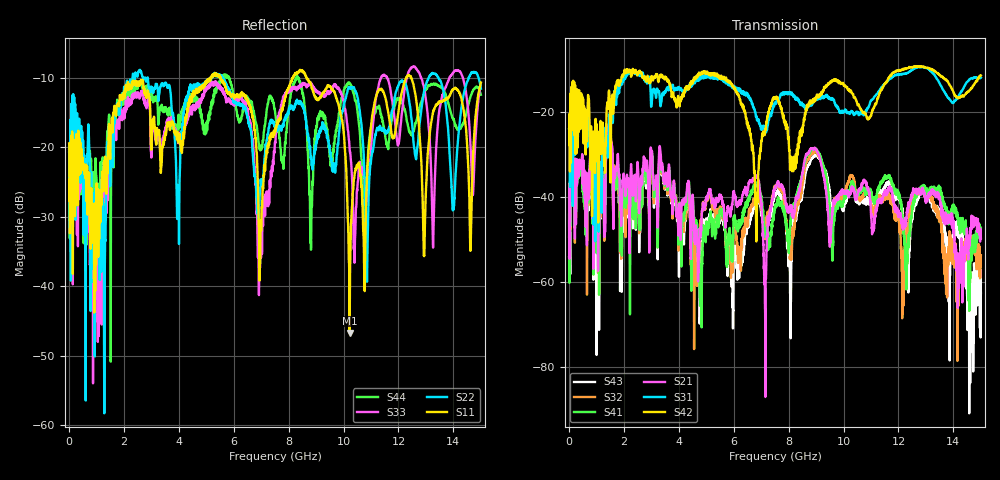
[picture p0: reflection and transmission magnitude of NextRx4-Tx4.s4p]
! FILE: N:\QM 2007\Prüfprotokolle\Highspeed\Konfektionierte Ltg\L45593-D106\D30\8216\0002\Next  Platine 2\NextRx4-Tx4.s4p
# MHz S DB R 50.00
! FREQ  S11  S12  S13  S14
!  S21  S22  S23  S24
!  S31  S32  S33  S34
!  S41  S42  S43  S44
!  DB  ANG  DB  ANG  DB  ANG  DB  ANG
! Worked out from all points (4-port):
!   2999 points, 10 MHz to 15 GHz, reference 50 ohm
!   strongest paths, dB at 10 MHz, 3.755 GHz, 7.505 GHz, 11.26 GHz, 15 GHz:
!     S42: -23.9, -15.9, -16.9, -16.7, -11.3
!     S31: -24.0, -13.7, -18.1, -15.2, -11.8
!     S21: -45.7, -39.4, -37.7, -40.6, -49.7
!     S41: -44.1, -38.8, -41.9, -38.2, -47.1
!     S32: -49.3, -38.7, -37.7, -39.9, -53.7
!     S43: -54.1, -39.3, -39.1, -40.3, -62.6
!   lowest |S11| = -46.7 dB at 10.22 GHz (marker M1), VSWR 1.01, Z = 49.7 + j0.3 ohm
!   |S11| at or under -10 dB: start of sweep to 5.159 GHz; 5.533 GHz to 8.151 GHz (2.618 GHz wide, 38.3 % of centre); 8.648 GHz to 12.28 GHz (3.634 GHz wide, 34.7 % of centre)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
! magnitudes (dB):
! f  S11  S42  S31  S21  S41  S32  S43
! 10 MHz  -19.4  -23.9  -24.0  -45.7  -44.1  -49.3  -54.1
! 1.485 GHz  -20.0  -16.6  -20.9  -22.1  -22.7  -21.8  -22.8
! 4.795 GHz  -11.3  -11.1  -12.1  -47.4  -60.0  -45.3  -53.3
! 6.94 GHz  -39.2  -30.6  -22.4  -38.0  -37.7  -40.6  -40.8
! 8.47 GHz  -9.1  -25.1  -17.9  -35.7  -35.2  -39.1  -40.0
! 10.22 GHz  -46.7  -15.0  -20.2  -39.0  -38.3  -35.6  -38.9
! 15 GHz  -10.7  -11.3  -11.8  -49.7  -47.1  -53.7  -62.6
